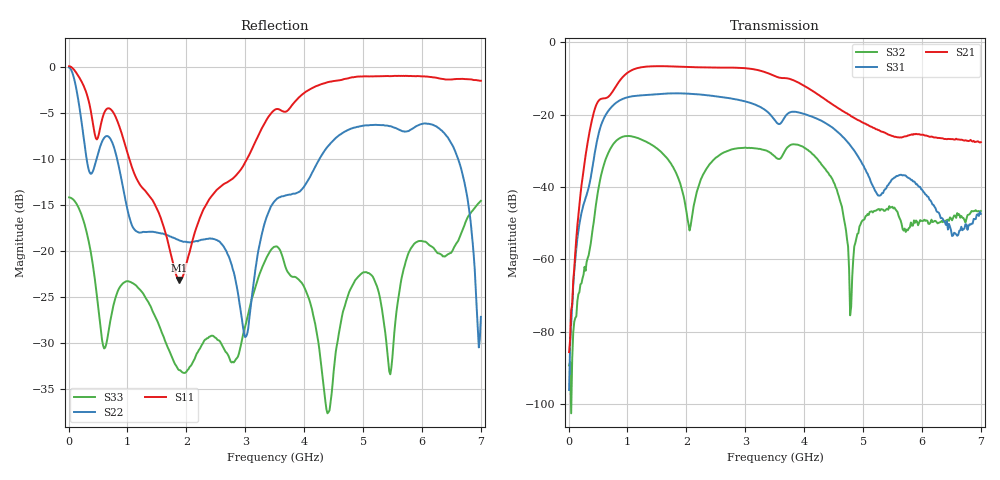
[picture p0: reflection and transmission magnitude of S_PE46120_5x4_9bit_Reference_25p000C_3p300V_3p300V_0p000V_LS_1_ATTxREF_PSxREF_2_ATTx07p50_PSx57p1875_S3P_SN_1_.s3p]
! Device ID: PE46120_5x4_9bit_Reference
! Device ID: PE46120_5x4_9bit_Reference
! File Path: z:\PE46120_5x4_9bit_Reference\MPAC_Yi\new_12port\25p000C\3p300\LS_1_ATTxREF_PSxREF_2_ATTx07p50_PSx57p1875\PE46120_5x4_9bit_Reference_25p000C_3p300V_3p300V_0p000V_LS_1_ATTxREF_PSxREF_2_ATTx07p50_PSx57p1875_S3P_SN_1_.s3p
! Serial: 1
! Lot:
! Temp: 25.000C
! VDD: 3.300
! VSS: 0.000
! Control_Hi: 3.300
! Control_Lo: 0.000
! Logic State: LS_1_ATTxREF_PSxREF_2_ATTx07p50_PSx57p1875
! Port 1: RFin
! Port 2: RFout1
! Port 3: RFout2
! ThroughPath:1-3
! IDD: -0.000542247
! ISS: 0
! Comment:
#  Hz  S  RI  R  50
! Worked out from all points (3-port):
!   401 points, 10 MHz to 7 GHz, reference 50 ohm
!   strongest paths, dB at 10 MHz, 1.758 GHz, 3.505 GHz, 5.253 GHz, 7 GHz:
!     S21: -85.7, -6.6, -9.3, -24.2, -27.6
!     S31: -96.2, -14.1, -21.6, -42.3, -47.4
!     S32: -89.4, -34.1, -31.6, -46.2, -46.6
!   lowest |S11| = -23.2 dB at 1.88 GHz (marker M1), VSWR 1.15, Z = 57.2 + j1.71 ohm
!   |S11| at or under -10 dB: 1.031 GHz to 3.031 GHz (2 GHz wide, 98.5 % of centre)
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1e7  1 -0.1155  -3.96e-05 -0.000117  -1.2e-05 0.000181
     2e-05 -4.79e-05  0.9858 -0.0969  1.05e-05 1.21e-05
     1.54e-05 -2.33e-06  -2.31e-05 2.49e-05  0.1948 -0.00819
2.37175e8  -0.4748 -0.6587  -0.0124 -0.00523  -0.00445 0.00196
           -0.0123 -0.00515  -0.2945 -0.3534  -0.000178 0.00063
           -0.00461 0.00197  -0.00016 0.000519  0.0911 -0.1208
4.6435e8  -0.403 -0.0647  -0.0596 0.1162  -0.03 0.0196
          -0.0604 0.118  0.1375 0.2737  0.00198 -0.00523
          -0.0303 0.0197  0.00189 -0.00529  -0.0281 -0.0568
9.36175e8  -0.2553 0.3078  0.3377 -0.0282  0.1613 -0.0372
           0.3413 -0.0288  -0.0466 -0.2057  0.049 0.0046
           0.1633 -0.0379  0.0498 0.00459  0.0571 0.035
1.879825e9  0.0678 0.0148  -0.433 0.1472  -0.1882 0.0514
            -0.4377 0.1495  -0.1096 0.0308  0.00714 0.00982
            -0.1905 0.0523  0.00737 0.00968  0.0213 -0.00688
3.505e9  -0.4596 -0.3604  -0.0804 -0.3277  -0.00664 -0.0818
         -0.0811 -0.3319  0.0648 0.1754  -0.025 0.0066
         -0.00717 -0.083  -0.0256 0.00673  0.0527 0.0911
4.44865e9  -0.8262 -0.0856  -0.0517 0.1332  -0.0322 0.0603
           -0.0517 0.1353  -0.3832 -0.0211  0.0131 -0.00458
           -0.0325 0.0611  0.0132 -0.00499  0.00445 0.0144
4.79815e9  -0.8664 0.1098  0.0283 0.0905  0.0195 0.0296
           0.0289 0.0905  -0.3207 0.3312  0.000281 0.000269
           0.02 0.0302  -1.99e-05 0.00022  0.0436 0.0453
5.1127e9  -0.8312 0.3059  0.0495 0.0481  0.012 0.00521
          0.0503 0.0483  -0.0533 0.4784  0.00152 0.00398
          0.0122 0.00503  0.00188 0.00411  0.0736 -0.0146
7e9  -0.0868 0.8343  -0.0229 -0.0335  0.00421 -0.00117
     -0.0229 -0.0349  -0.0368 0.0236  0.00166 0.00449
     0.00409 -0.00121  0.00143 0.00443  0.1149 0.1472
